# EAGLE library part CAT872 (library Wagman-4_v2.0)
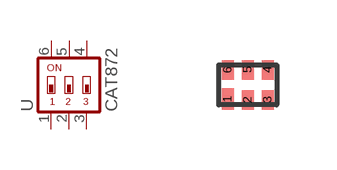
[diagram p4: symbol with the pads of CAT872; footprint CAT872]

Designator prefix -

## CAT872  [CAT872]
1  1  pas
2  2  pas
3  3  pas
4  4  pas
5  5  pas
6  6  pas

## Footprint CAT872 (pad centres in mm)
smd 0.3 x 0.53: 1 -0.5,-0.355
smd 0.3 x 0.49: 2 0,-0.375; 3 0.5,-0.375; 4 0.5,0.375; 5 0,0.375; 6 -0.5,0.375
